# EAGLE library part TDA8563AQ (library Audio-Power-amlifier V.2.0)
The TDA8563AQ is an integrated class-B output amplifier in a 13-lead single-in-line (SIL) power package. It contains 2 ´ 40 W/2 W amplifiers in a BTL configuration.
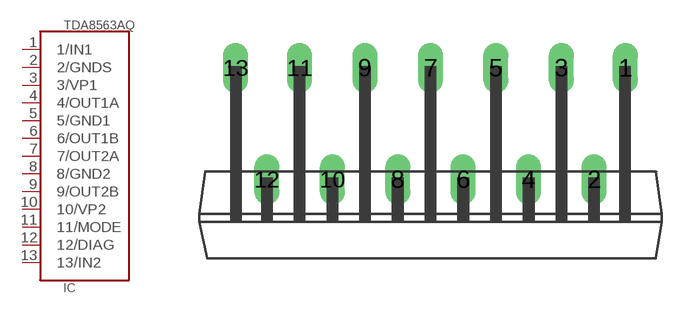
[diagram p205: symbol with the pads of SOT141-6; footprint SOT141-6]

Designator prefix IC

## TDA8563AQ  [SOT141-6]
1  1/IN1  in
2  2/GNDS  pwr
3  3/VP1  pwr
4  4/OUT1A  out
5  5/GND1  pwr
6  6/OUT1B  out
7  7/OUT2A  out
8  8/GND2  pwr
9  9/OUT2B  out
10  10/VP2  pwr
11  11/MODE  in
12  12/DIAG  out
13  13/IN2  in

## Footprint SOT141-6 (pad centres in mm)
drill 0.8 long: 1 10.12,5.8; 2 8.5,0; 3 6.8,5.8; 4 5.1,0; 5 3.4,5.8; 6 1.7,0; 7 0,5.8; 8 -1.7,0; 9 -3.4,5.8; 10 -5.1,0; 11 -6.8,5.8; 12 -8.5,0; 13 -10.12,5.8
